FUNCTION_BLOCK FB_File
VAR
	fbFileStream : FB_ALYC_FileStream;
	
	bStart : BOOL := FALSE;
	bStop : BOOL := FALSE;	
	bReconfigure : BOOL := FALSE;
	
	stFileConfig : ST_ALYC_FileStreamConfig := (
		bAutostartStream:=TRUE,
		nSamplingDivider:=2,
		nAdsBuffer:=20,
		sFileDir:='%TC_BOOTPRJPATH%',
		nMaxFileSize := 10,
		bEnableRingBuffer := TRUE,
		nFilesInRingBuffer := 4,
		stDeviceLocation:=(sAddress:='TheNewAddress', sLatitude:='TheNewLatitude', sLongitude:='TheNewLongitude'));
END_VAR

IF fbFileStream.bInitialized THEN
	IF bStart THEN
		bStart := FALSE;
		fbFileStream.Start();
	ELSIF bStop THEN
		bStop := FALSE;
		fbFileStream.Stop();
	END_IF

	IF bReconfigure THEN
		fbFileStream.Reconfigure(stFileConfig);
		IF fbFileStream.eReconfigState = E_ALYC_ReconfigState.DONE THEN
			bReconfigure := FALSE;
		ELSE
			RETURN;
		END_IF
	END_IF	
END_IF

END_FUNCTION_BLOCK
